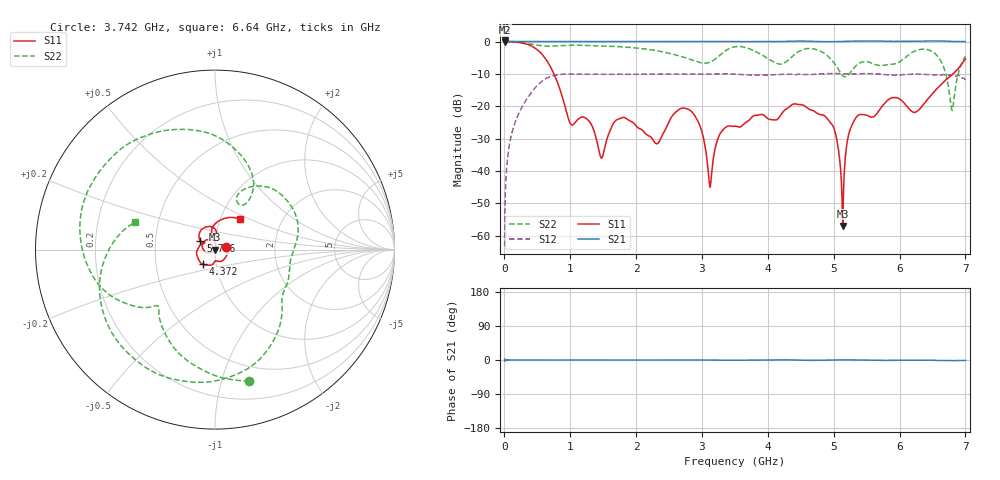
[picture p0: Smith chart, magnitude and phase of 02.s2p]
!Keysight Technologies,N5232A,MY52221221,A.10.65.11
!Date: Wednesday, October 16, 2024 11:49:55
!Correction: S11(Full 2 Port(1,4))
!S41(Full 2 Port(1,4))
!S14(Full 2 Port(1,4))
!S44(Full 2 Port(1,4))
!S2P File: Measurements: S11, S41, S14, S44:
# Hz S  RI  R 50
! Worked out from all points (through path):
!   4000 points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, 2.05 MHz to 7 GHz, reference 50 ohm
!   highest |S21| = 0.33 dB at 2.05 MHz (marker M1); lowest = -0.2 dB at 5.55 MHz (marker M2)
!   lowest |S11| = -57.0 dB at 5.136 GHz (marker M3), VSWR 1.00, Z = 50.1 - j0.0739 ohm
!   |S11| at or under -10 dB: 751 MHz to 6.814 GHz (6.063 GHz wide, 160 % of centre)
!   |S22| runs from -21.2 to 0.0 dB; largest |S21 - S12| = 1.3
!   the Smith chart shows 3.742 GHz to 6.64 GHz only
!   S11 on the Smith chart (normalised r, x): 3.742 GHz: 1.14, +0.03; 4.372 GHz: 0.86, -0.14; 5.716 GHz: 0.85, +0.08; 6.64 GHz: 1.24, +0.44
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2049925  -0.97 0.1502  1.038 0.0239  0.000119 0.000677  -0.9783 0.097
5549775  -1.002 0.0473  0.9748 0.0301  0.000117 0.00192  -1.003 0.0188
1.822922e8  -0.022 0.9773  0.999 0.000242  0.0611 0.0193  -0.8112 0.549
3.415354e8  0.8928 0.1653  0.9997 -0.000455  0.0873 -0.098  -0.4305 0.8301
6.320229e8  -0.4592 -0.2586  0.9993 -0.0014  -0.2683 0.0104  0.2718 0.8055
1.16925e9  0.0317 0.06  0.9985 -2.29e-05  0.1623 -0.2666  0.8443 -0.2238
1.687228e9  0.0597 0.000876  0.9994 -0.00175  -0.0317 0.31  -0.1313 -0.8274
2.3347e9  -0.00226 0.0271  0.9991 -0.00139  -0.2862 -0.1284  -0.6349 0.3264
2.814179e9  0.0763 -0.0424  1.002 0.000376  0.2975 0.1011  0.117 0.5198
3.123916e9  0.00221 -0.00519  1.006 -0.00293  -0.0567 -0.3086  0.3159 0.3606
3.5019e9  -0.0481 0.00974  1 -0.0115  -0.1206 0.2879  0.7871 -0.2641
3.74164e9  0.0639 0.0127  0.9961 -0.00563  0.2822 0.1088  0.1906 -0.7314
4.371613e9  -0.0681 -0.0815  1.012 0.00251  -0.2399 0.2  -0.5063 -0.2963
4.66735e9  -0.0828 0.0265  1.005 -0.0161  0.2754 0.1402  -0.6079 0.4794
5.13633e9  0.0012 -0.000737  1.002 0.00447  -0.2897 -0.1309  0.1616 0.2495
5.290323e9  -0.0534 -0.0106  1.01 0.00227  -0.2566 0.1825  0.1586 0.3341
5.715555e9  -0.0815 0.0463  1.014 -0.017  0.2892 -0.121  0.4203 -0.0603
5.83455e9  -0.0859 0.094  1.006 -0.0163  0.1116 -0.283  0.4089 -0.1657
6.30703e9  -0.0171 0.0888  1.01 -0.00844  -0.0818 0.3028  -0.1565 -0.7351
6.639515e9  0.1404 0.1706  1.017 -0.0257  0.2649 -0.1502  -0.448 0.1512
6.798759e9  0.2895 -0.0988  1.004 -0.0298  -0.0457 -0.3071  -0.0865 -0.00391
7e9  -0.4444 -0.3032  0.9988 -0.0201  -0.2491 0.0591  -0.5879 -0.0426
